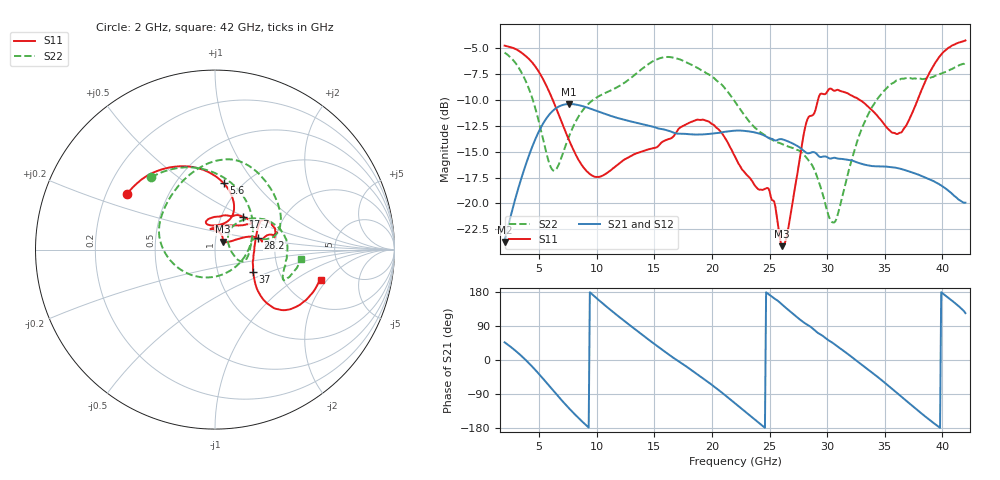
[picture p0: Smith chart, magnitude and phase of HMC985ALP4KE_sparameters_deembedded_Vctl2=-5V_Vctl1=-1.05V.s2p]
!s2p File: Measurements: S11, S21, S12, S22
# GHz S dB R 50.0
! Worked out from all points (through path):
!   401 points, 2 GHz to 42 GHz, reference 50 ohm
!   highest |S21| = -10.38 dB at 7.6 GHz (marker M1); lowest = -23.7 dB at 2 GHz (marker M2)
!   lowest |S11| = -24.1 dB at 26.1 GHz (marker M3), VSWR 1.13, Z = 54.4 + j4.74 ohm
!   |S11| at or under -10 dB: 6.186 GHz to 29.2 GHz (23.01 GHz wide, 130 % of centre); 32.84 GHz to 37.85 GHz (5.011 GHz wide, 14.2 % of centre)
!   |S22| runs from -21.8 to -5.4 dB; largest |S21 - S12| = 0.0003
!   S11 on the Smith chart (normalised r, x): 2 GHz: 0.29, +0.27; 5.6 GHz: 0.82, +0.71; 17.7 GHz: 1.27, +0.49; 28.2 GHz: 1.61, +0.22; 37 GHz: 1.48, -0.39; 42 GHz: 3.17, -1.73
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2  -4.73 147.7  -23.73 46.6  -23.73 46.6  -5.40 131.4
3.6  -5.53 121.2  -17.05 6.8  -17.05 6.8  -7.62 86.7
4.7  -6.80 100.2  -13.70 -27.3  -13.70 -27.3  -10.93 44.8
5.6  -8.55 82.7  -11.81 -58.6  -11.82 -58.6  -15.01 -6.7
6.4  -10.58 70.1  -10.84 -87.0  -10.84 -87.0  -16.79 -72.9
7.6  -13.90 63.1  -10.38 -127.7  -10.38 -127.7  -13.48 -144.5
8.7  -16.30 71.6  -10.56 -161.4  -10.57 -161.4  -11.11 -176.0
12  -16.09 108.7  -11.79 112.4  -11.80 112.5  -8.61 136.8
15.4  -14.38 79.0  -12.76 33.4  -12.77 33.4  -5.98 85.6
17.7  -12.38 49.1  -13.27 -15.5  -13.27 -15.4  -6.30 58.4
19.9  -12.24 36.4  -13.25 -63.5  -13.26 -63.4  -7.64 28.3
22  -15.46 53.0  -12.96 -114.3  -12.96 -114.3  -10.16 11.5
24.9  -18.55 97.0  -13.66 173.9  -13.67 174.0  -13.62 11.3
26.1  -24.13 44.2  -13.79 146.0  -13.80 146.1  -14.26 -1.7
28.2  -12.15 15.2  -15.10 94.5  -15.10 94.6  -15.57 -23.7
28.7  -11.49 9.9  -15.04 84.3  -15.05 84.3  -16.31 -24.6
30.6  -9.10 16.5  -15.58 42.4  -15.58 42.4  -21.84 20.5
33  -10.10 31.7  -16.18 -12.3  -16.18 -12.3  -12.78 46.2
35.4  -12.90 9.4  -16.46 -70.1  -16.47 -70.0  -8.61 20.0
37  -12.17 -30.4  -16.86 -111.0  -16.86 -110.9  -7.88 1.4
39.6  -6.04 -42.4  -18.06 -174.5  -18.06 -174.4  -7.60 -23.8
42  -4.23 -16.0  -19.93 123.7  -19.93 123.7  -6.38 -6.1
